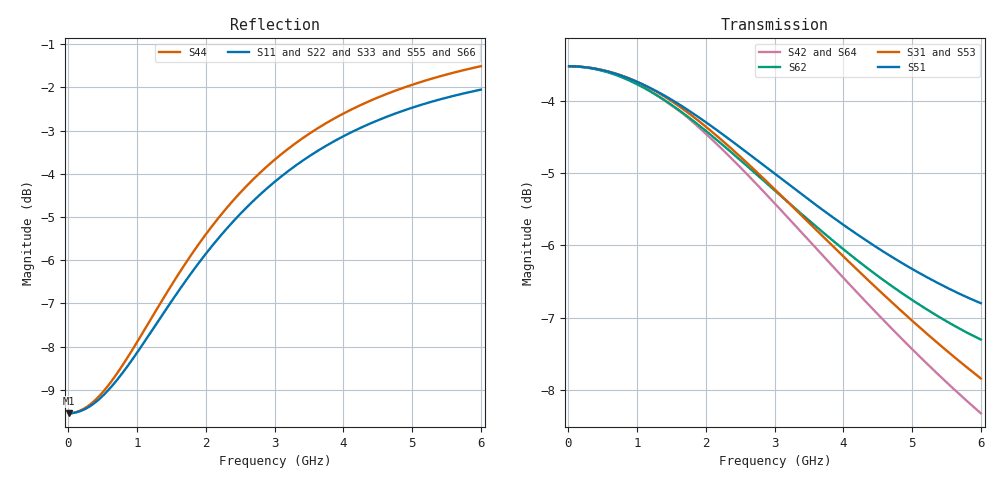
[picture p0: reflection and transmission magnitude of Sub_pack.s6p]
! Touchstone file from project Driver_Package_Study1
! Exported from HFSS 2015.1.0
! Variables:
!  BW_Xoffset = 0mm
!  BW_Yoffset = 0mm
!  BW_Zoffset = 0mm
!  FlangeL = 8.5mm
!  FlangeW = 4.9mm
!  LeadH = 1.05mm
!  Lg2_BG = 90um
!  Lg2_ED = 453um
!  Lg2_LH = 600um
!  Lg2_SP = 1000um
!  Lg2_X1 = 440um
!  Lg2_X2 = 531um
!  Lg2_X3 = 631um
!  Lg2_X4 = 738um
!  Lg2_XX = 700um
!  Lg2_YY = -2550um
!  Lg2_Z1 = 568.2um
!  Lg2_Z2 = 608.4um
!  Lg2_Z3 = 603.6um
!  Lg2_Z4 = 566.4um
!  PCB_bot = -1.368mm
!  PCB_metalT = 60um
!  PCB_t = 0.508mm
!  PCB_top = -0.86mm
!  PCB_x = 10mm
!  baseplate_x = 26.4mm
!  bot = -0.8mm
!  deem_x = 9.2mm
!  gap = 100um
!  heatsink_x = 6.2mm
!  heatsink_y = 40mm
!  lead_bot = -0.86mm
!  lead_ext_ref = 4mm
!  lead_w = 4.95mm
!  via_x = 5.6mm
!  via_y = 10mm
# GHZ S MA R 50.000000
! Terminal data exported
! Port[1] = Lead_in_internal
! Port[2] = Lead_out_internal
! Port[3] = Lead_in_c
! Port[4] = Lead_out_c
! Port[5] = Lead_in
! Port[6] = Lead_out
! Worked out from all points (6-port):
!   600 points, 10 MHz to 6 GHz, reference per port
!   strongest paths, dB at 10 MHz, 1.51 GHz, 3.01 GHz, 4.51 GHz, 6 GHz:
!     S51: -3.5, -4.0, -5.0, -6.0, -6.8
!     S31: -3.5, -4.0, -5.2, -6.6, -7.8
!     S62: -3.5, -4.1, -5.2, -6.4, -7.3
!     S53: -3.5, -4.1, -5.3, -6.7, -8.0
!     S42: -3.5, -4.1, -5.4, -7.0, -8.3
!     S64: -3.5, -4.1, -5.5, -7.0, -8.4
!   lowest |S11| = -9.5 dB at 10 MHz (marker M1), VSWR 2.00
!   |S11| at or under -10 dB: nowhere
